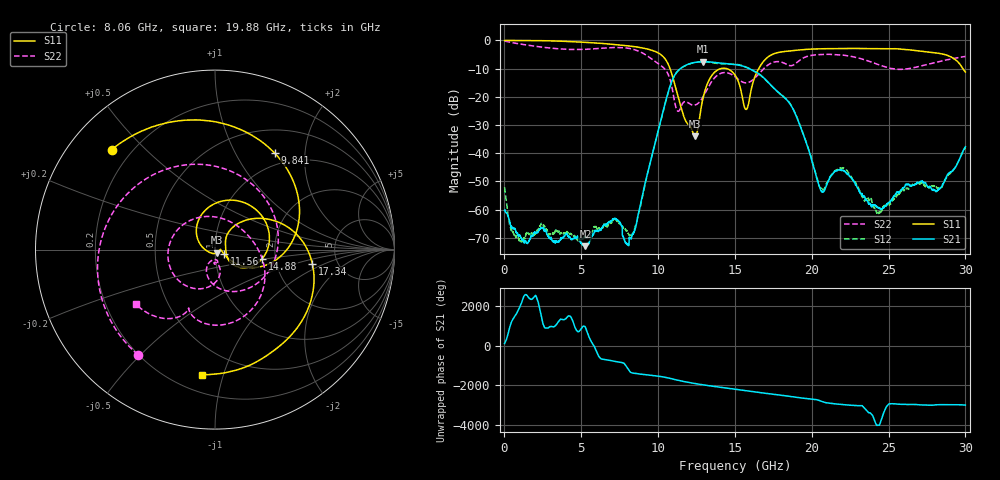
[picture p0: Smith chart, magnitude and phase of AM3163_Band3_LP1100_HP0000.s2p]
!Agilent Technologies,E8364B,MY43040894,A.07.50.67
!Agilent E8364B: A.07.50.67
!Date: Thursday, August 20, 2020 12:11:31
!Correction: S11(Full 2 Port(1,2))
!S21(Full 2 Port(1,2))
!S12(Full 2 Port(1,2))
!S22(Full 2 Port(1,2))
!S2P File: Measurements: S11, S21, S12, S22:
# Hz S  dB  R 50
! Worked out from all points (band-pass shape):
!   3201 points, 10 MHz to 30 GHz, reference 50 ohm
!   highest |S21| = -7.53 dB at 12.93 GHz (marker M1); lowest = -73.0 dB at 5.268 GHz (marker M2)
!   |S21| within 3 dB of the highest: 11.34 GHz to 16.13 GHz (4.797 GHz wide, 34.9 % of centre)
!   lowest |S11| = -33.9 dB at 12.39 GHz (marker M3), VSWR 1.04, Z = 51.1 - j1.71 ohm
!   |S11| at or under -10 dB: 10.78 GHz to 14.08 GHz (3.302 GHz wide, 26.6 % of centre); 14.47 GHz to 16.55 GHz (2.074 GHz wide, 13.4 % of centre); 29.83 GHz to end of sweep
!   |S22| runs from -25.1 to -0.2 dB; largest |S21 - S12| = 0.014
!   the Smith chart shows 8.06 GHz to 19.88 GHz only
!   S11 on the Smith chart (normalised r, x): 8.06 GHz: 0.13, +0.40; 9.841 GHz: 0.82, +1.46; 11.56 GHz: 1.10, -0.06; 14.88 GHz: 1.70, -0.19; 17.34 GHz: 3.24, -0.75; 19.88 GHz: 0.31, -0.85
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1e7  -0.01 -2.2  -60.25 120.6  -52.06 43.1  -0.23 -5.9
1.153369e9  -0.00 -31.6  -70.82 120.3  -71.36 161.3  -1.39 -83.6
2.521662e9  -0.09 -69.1  -66.34 13.0  -65.38 55.3  -2.43 -165.4
5.014581e9  -0.61 -135.6  -71.82 175.5  -70.26 -148.6  -3.20 62.1
5.267622e9  -0.68 -142.3  -72.98 -127.4  -70.08 -31.1  -3.16 48.2
6.560941e9  -1.14 -177.8  -65.22 25.3  -65.71 17.8  -2.69 -26.9
8.060441e9  -1.92 136.0  -72.42 -98.9  -68.40 -41.9  -2.78 -126.2
9.841097e9  -3.98 58.3  -35.65 -79.2  -35.64 -79.7  -7.58 59.7
1.000979e10  -4.43 47.7  -31.99 -97.1  -32.02 -97.4  -8.24 35.9
1.155615e10  -24.96 -26.9  -9.57 11.4  -9.60 11.5  -22.70 -77.9
1.239025e10  -33.94 -56.3  -7.79 -109.0  -7.82 -108.9  -22.91 -88.2
1.293382e10  -20.20 155.4  -7.53 -177.3  -7.56 -177.7  -19.96 -75.4
1.378666e10  -10.78 72.5  -7.86 87.0  -8.12 87.0  -12.66 -110.2
1.488317e10  -11.44 -10.9  -8.48 -24.7  -8.44 -22.8  -12.39 156.2
1.5005e10  -12.27 -19.2  -8.55 -37.2  -8.46 -35.5  -12.86 143.8
1.574538e10  -24.44 9.2  -9.55 -115.0  -9.45 -115.0  -15.04 64.2
1.73386e10  -5.21 -8.5  -15.83 79.4  -15.95 80.6  -8.09 -60.0
1.987838e10  -3.09 -96.1  -40.14 -166.3  -40.05 -167.2  -5.41 -145.6
2.000958e10  -3.06 -99.5  -42.74 -177.0  -42.39 -179.0  -5.27 -150.5
2.277428e10  -2.84 -163.4  -50.30 -146.1  -50.15 -147.5  -5.88 107.3
2.500479e10  -2.98 144.2  -57.72 -78.4  -58.68 -54.3  -9.77 -10.3
3e10  -11.20 -31.2  -37.71 -123.7  -38.03 -118.5  -5.70 116.5
